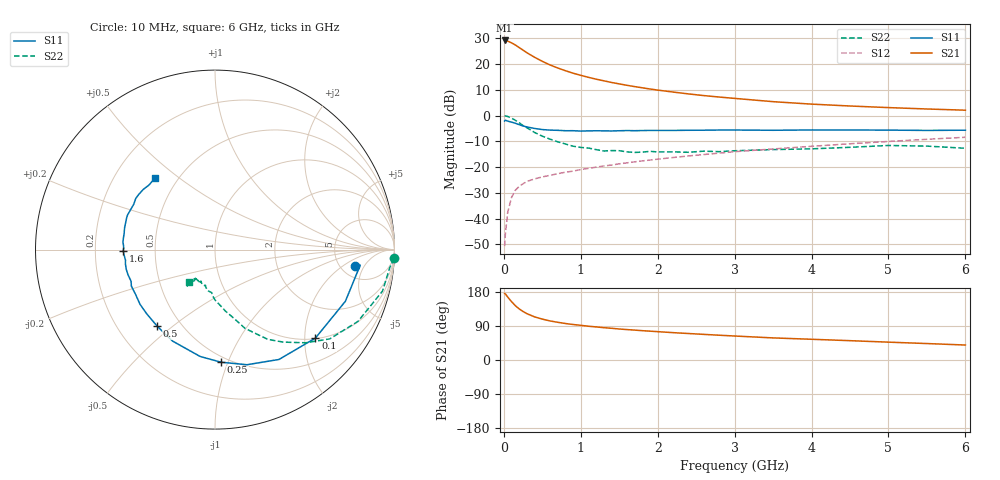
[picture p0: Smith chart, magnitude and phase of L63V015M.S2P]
!  INFINEON TECHNOLOGIES Small Signal Semiconductors
! BFR380L3 , Si-NPN RF-Transistor in TSLP-3-1
!  Vce=3 V,  Ic=15 mA
! Common Emitter S-Parameters:  07. March 2005
#  GHz  S  MA  R  50
! f  S11  S21  S12  S22
! GHz  Mag  Ang  Mag  Ang  Mag  Ang  Mag  Ang
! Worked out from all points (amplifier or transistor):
!   36 points, 10 MHz to 6 GHz, reference 50 ohm
!   highest |S21| = 29.2 dB at 10 MHz (marker M1)
!   |S21| within 3 dB of that: start of sweep to 211.5 MHz
!   unconditionally stable (mu >= 1): 1.975 GHz to 4.784 GHz
!   at 250 MHz: K = 0.32, MSG = 26.0 dB, |S12| = -26.5 dB
!   at 1.4 GHz: K = 0.93, MSG = 16.0 dB, |S12| = -19.2 dB
!   at 6 GHz: K = 0.97, MSG = 5.3 dB, |S12| = -8.4 dB
!   S11 on the Smith chart (normalised r, x): 10 MHz: 6.68, -3.22; 100 MHz: 1.02, -2.26; 250 MHz: 0.46, -0.95; 500 MHz: 0.37, -0.44; 1.6 GHz: 0.32, -0.01; 6 GHz: 0.38, +0.41
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0.01  0.7842 -6.8  28.82 175.3  0.0029 80.6  1.001 -2.8
0.02  0.8138 -6.1  28.66 174.5  0.005 89.9  0.9793 -5.8
0.05  0.7815 -21.6  27.97 166.2  0.0131 82.5  0.9616 -13.9
0.1  0.7457 -41.4  25.91 154.0  0.0256 71.7  0.8912 -26.7
0.15  0.7083 -59.8  23.51 143.3  0.0355 63.6  0.81 -37.9
0.2  0.6656 -74.5  20.94 134.7  0.0421 59.7  0.7243 -45.8
0.25  0.6284 -86.9  18.69 128.0  0.0474 55.2  0.6403 -53.6
0.3  0.6012 -97.9  16.63 122.2  0.0524 52.8  0.5806 -59.5
0.4  0.5618 -114.9  13.57 113.8  0.0589 50.4  0.4701 -69.1
0.5  0.5346 -127.1  11.33 107.9  0.0643 50.1  0.3981 -74.5
0.6  0.5221 -136.8  9.631 103.1  0.069 50.3  0.3489 -80.2
0.7  0.5171 -143.9  8.414 99.5  0.0742 51.0  0.3092 -85.1
0.9  0.5085 -156.4  6.657 93.7  0.0833 53.1  0.2539 -93.4
1.1  0.5046 -163.9  5.533 89.1  0.0942 54.9  0.234 -98.9
1.4  0.5022 -173.3  4.401 83.7  0.1093 57.6  0.2089 -105.7
1.6  0.5117 -179.2  3.876 80.3  0.1206 58.6  0.197 -113.6
2.2  0.5144 169.7  2.864 72.2  0.1531 60.9  0.1972 -118.2
2.8  0.5235 159.9  2.291 65.4  0.1864 62.3  0.1989 -125.6
3.5  0.5182 151.0  1.863 58.3  0.2246 61.4  0.2184 -126.2
4.5  0.5244 144.2  1.535 51.0  0.2833 61.2  0.2417 -127.1
5.5  0.5145 135.7  1.343 43.4  0.3459 58.4  0.2551 -127.7
6  0.5199 130.3  1.272 39.5  0.379 56.6  0.2316 -129.4
